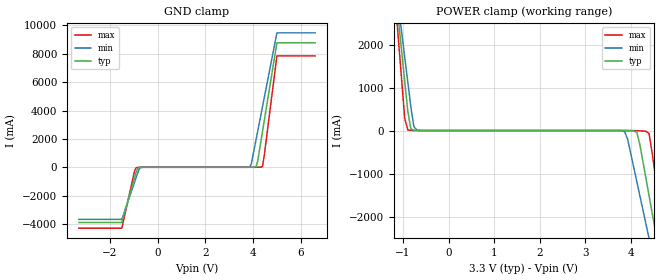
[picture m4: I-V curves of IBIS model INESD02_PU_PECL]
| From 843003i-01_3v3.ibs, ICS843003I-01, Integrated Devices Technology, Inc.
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[Model]   INESD02_PU_PECL
Model_type  Input
Polarity   Non-Inverting
Vinl = 0.8V
Vinh = 2.0V
|   typ   min   max
C_comp   2pF   1.5pF   2.5pF
|   typ   min   max
[Voltage range]  3.3V   3.15V   3.45V
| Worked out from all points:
|   GND clamp passes 1 mA (typ) near -0.59 V on its own axis
|   POWER clamp passes 1 mA (typ) near -0.70 V on its own axis
[GND_clamp]
|Voltage   I(typ)   I(min)   I(max)
-3.3V     -3.894A    -3.674A    -4.294A
-1.5V     -3.894A    -3.674A    -4.294A
-963.9mV  -730.3mA   -1.043A    -249.9mA
-896.9mV  -335.4mA   -714.7mA   -27.07mA
-695.9mV  -3.401mA   -10.69mA   -6.477mA
3.861V    50.74uA    27.7mA     7.469uA
3.928V    181.1uA    239mA      10.12uA
4.129V    40.44mA    1.967A     268.6uA
4.196V    445.8mA    2.543A     887.9uA
4.397V    2.525A     4.275A     64.01mA
5V        8.773A     9.475A     7.854A
6.6V      8.773A     9.475A     7.854A
[POWER_clamp]
|Voltage   I(typ)   I(min)   I(max)
-3.3V     6.7A       6.327A     7.39A
-1.165V   3.23A      3.44A      2.951A
-1.031V   1.842A     2.286A     1.176A
-963.9mV  1.149A     1.709A     289.6mA
-896.9mV  456.4mA    1.132A     15.33mA
-695.9mV  727.9uA    10.66mA    491.6uA
3.861V    -620.9uA   -26.2mA    -103.4uA
4.129V    -41.91mA   -1.19A     -4.968mA
4.33V     -1.119A    -2.176A    -17.93mA
4.531V    -2.305A    -3.163A    -1.019A
4.732V    -3.492A    -4.151A    -2.536A
6.6V      -5.075A    -5.469A    -4.558A
